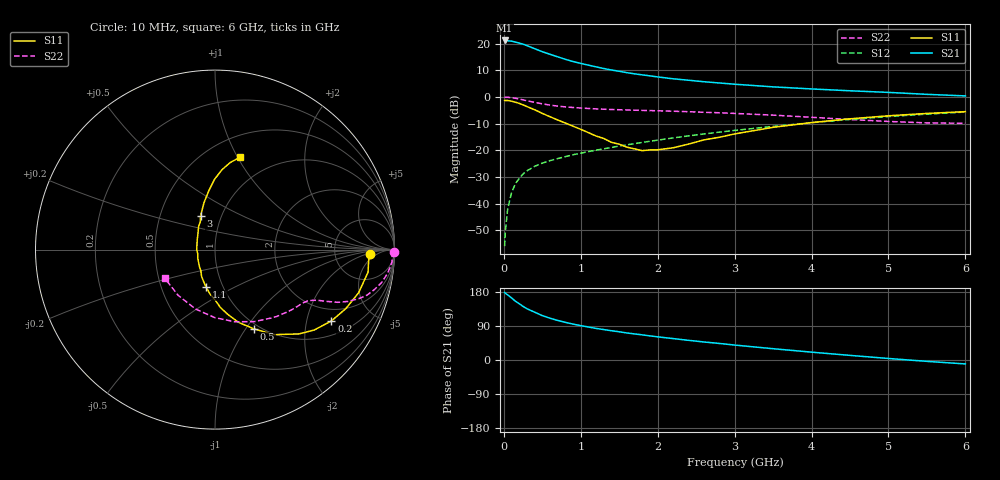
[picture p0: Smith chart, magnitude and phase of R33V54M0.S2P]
! SIEMENS Small Signal Semiconductors
! BFR181
! Si NPN RF Bipolar Junction Transistor in SOT23
! VCE = 3.5 V  IC = 4 mA
! Common Emitter S-Parameters:  May  1996
# GHz  S  MA  R  50
!  f  S11  S21  S12  S22
! GHz  MAG  ANG  MAG  ANG  MAG  ANG  MAG  ANG
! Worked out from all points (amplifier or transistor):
!   36 points, 10 MHz to 6 GHz, reference 50 ohm
!   highest |S21| = 21.2 dB at 10 MHz (marker M1)
!   |S21| within 3 dB of that: start of sweep to 392.5 MHz
!   unconditionally stable (mu >= 1): 1.235 GHz to 3.065 GHz
!   at 250 MHz: K = 0.36, MSG = 24.3 dB, |S12| = -28.8 dB
!   at 1.4 GHz: K = 1.04, MAG = 13.3 dB, |S12| = -18.9 dB
!   at 6 GHz: K = 0.86, MSG = 3.0 dB, |S12| = -5.6 dB
!   S11 on the Smith chart (normalised r, x): 10 MHz: 13, -3; 200 MHz: 1.50, -2.82; 500 MHz: 0.94, -1.10; 1.1 GHz: 0.83, -0.36; 3 GHz: 0.80, +0.31; 6 GHz: 0.71, +1.02
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0.01  0.8637 -1.8  11.49 178.2  0.0016 92.4  0.995 -0.7
0.02  0.8583 -3.4  11.39 176.3  0.0031 87.5  0.9876 -1.6
0.05  0.8619 -8.4  11.32 171.7  0.008 85.1  0.9887 -4.0
0.1  0.8357 -16.7  11.16 163.8  0.016 81.2  0.9722 -7.6
0.15  0.7994 -24.3  10.72 155.2  0.0237 75.9  0.9463 -11.2
0.2  0.7607 -31.5  10.26 148.5  0.0299 74.4  0.9164 -14.0
0.25  0.7117 -39.0  9.791 141.4  0.0361 70.5  0.8851 -16.6
0.3  0.6632 -45.1  9.195 135.4  0.0413 68.2  0.8511 -18.6
0.4  0.5778 -55.1  8.054 126.2  0.0502 64.7  0.7949 -21.3
0.5  0.4932 -63.7  7.07 117.1  0.0576 62.9  0.7455 -23.2
0.6  0.4273 -71.9  6.327 110.3  0.0642 61.7  0.7055 -24.3
0.7  0.3715 -78.4  5.672 104.4  0.0702 61.1  0.6752 -25.2
0.8  0.3247 -84.6  5.093 99.3  0.0764 60.7  0.6531 -25.8
0.9  0.2837 -89.4  4.625 94.7  0.0828 60.8  0.6363 -26.4
1.1  0.2145 -103.5  3.958 87.0  0.0947 61.4  0.61 -27.6
1.6  0.1148 -143.3  2.861 71.3  0.127 62.3  0.5712 -31.5
2.2  0.1117 152.8  2.198 56.5  0.171 61.5  0.5416 -38.4
3  0.2032 113.4  1.738 39.4  0.2365 57.6  0.4929 -50.7
3.5  0.2703 103.0  1.55 29.8  0.2817 53.9  0.4574 -61.3
4.5  0.3903 90.5  1.309 12.2  0.3804 44.1  0.3787 -90.3
5.5  0.4925 80.1  1.122 -3.6  0.4786 31.5  0.3273 -128.8
6  0.5318 75.0  1.049 -10.4  0.5231 24.5  0.3219 -150.0
